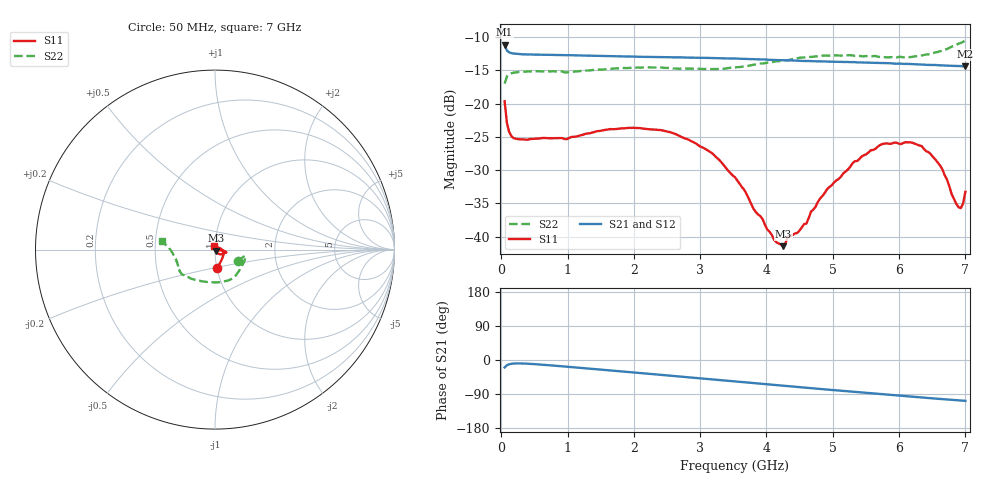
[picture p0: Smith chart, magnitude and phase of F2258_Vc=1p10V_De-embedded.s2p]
! Integrated Device Technology
! Corporate Headquarters
! 6024 Silver Creek Valley Road
! San Jose, CA 95138  USA
! Phone:  1-408-284-8200
! Toll Free:  1-800-223-1366
! Webpage:  http://www.idt.com/
! Timing and RF Division
! 515 Groton Road, Suite 102
! Westford, MA 01886-6024
! Device:  F2258
! Description: Voltage Variable RF Attenuator
! Frequency:  50.0 -  6000.00 MHz
! Package:  3x3 mm Thin QFN Plastic Package: 16 pin
! Ports:  2 RF, 2 DC
!  Pin  1  = NC
!  Pin  2  = NC
!  Pin  3  = RF2  = Port 2
!  Pin  4  = GND
!  Pin  5  = Vdd
!  Pin  6  = NC
!  Pin  7  = VCTRL
!  Pin  8  = NC
!  Pin  9  = GND
!  Pin 10  = RF1  = Port 1
!  Pin 11  = NC
!  Pin 12  = NC
!  Pin 13  = NC
!  Pin 14  = NC
!  Pin 15  = NC
!  Pin 16  = NC
! Vcntrl:  1.100 Volts
! Vdd:  +3.300 Volts
! Current:  1.162 mA
! Data:  The device was measured on a the F2258 evaluation board which has
!  individual transmission lines to the RF pins.  Data was collected
!  using a calibrated network analyzer.  The evaluation board was
!  de-embedded using a TRL calibration technique.
!  The reference plane is the edge of the package pin.
! Misc:  SN 10
!  Action Tracker AT0285
! Date Measured:  2014-12-10
! Date:  2016-01-13  MJV
! Note:
!  Integrated Device Technology supplies this data as a sample of measured
!  data at the package pin for this product.  Your particular data for this
!  product may vary.
!  Data was taken at 25 degrees C.
!  Integrated Device Technology reserves the right to change this data at anytime.
!Freq_(GHz)  S11M_(dB)  S11P_(deg)  S21M_(dB)  S21P_(deg)  S12M_(dB)  S12P_(deg)  S22M_(dB)  S22P_(deg)
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# GHz S dB R 50
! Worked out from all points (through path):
!   201 points, 50 MHz to 7 GHz, reference 50 ohm
!   highest |S21| = -11.14 dB at 50 MHz (marker M1); lowest = -14.4 dB at 7 GHz (marker M2)
!   group delay of S21, straight-line fit = 41.6 ps
!   lowest |S11| = -41.4 dB at 4.255 GHz (marker M3), VSWR 1.02, Z = 50.5 - j0.664 ohm
!   |S11| at or under -10 dB: start of sweep to end of sweep
!   |S22| runs from -17.0 to -10.5 dB; largest |S21 - S12| = 0.0014
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0.05  -19.62 -83.7  -11.14 -19.6  -11.13 -19.5  -16.98 -27.5
0.08475  -22.90 -61.4  -12.00 -13.9  -11.98 -13.9  -15.90 -15.4
0.189  -25.19 -31.2  -12.47 -9.3  -12.45 -9.3  -15.33 -11.1
1.2315  -24.67 -17.5  -12.77 -21.3  -12.75 -21.3  -15.04 -37.9
1.9265  -23.63 -14.3  -12.90 -31.8  -12.90 -31.8  -14.62 -55.5
2.37825  -23.96 -11.6  -12.98 -38.7  -12.99 -38.7  -14.55 -67.1
3.07325  -26.77 -8.1  -13.10 -49.6  -13.12 -49.6  -14.78 -89.5
3.525  -31.07 -8.1  -13.20 -56.8  -13.22 -56.7  -14.56 -107.3
4.11575  -40.48 -32.1  -13.43 -65.9  -13.38 -66.0  -13.68 -127.8
4.25475  -41.44 -50.8  -13.46 -68.0  -13.43 -68.1  -13.48 -131.1
4.32425  -40.00 -56.6  -13.48 -69.1  -13.44 -69.2  -13.47 -133.2
4.60225  -38.03 -67.0  -13.58 -73.3  -13.54 -73.3  -12.96 -139.0
4.7065  -35.92 -62.2  -13.61 -74.9  -13.55 -74.9  -12.94 -140.9
4.915  -32.85 -56.8  -13.66 -78.0  -13.61 -78.1  -12.77 -144.0
5.332  -28.65 -42.2  -13.75 -84.2  -13.74 -84.2  -12.82 -150.0
5.85325  -26.04 -26.6  -13.91 -91.7  -13.89 -91.8  -13.01 -159.8
6.20075  -25.88 -17.1  -14.05 -96.9  -14.03 -96.9  -12.96 -168.3
6.47875  -27.60 -4.0  -14.17 -100.8  -14.13 -100.8  -12.48 -175.6
6.6525  -29.86 10.0  -14.24 -103.2  -14.21 -103.2  -12.01 179.3
6.89575  -35.57 69.9  -14.34 -106.5  -14.33 -106.5  -10.97 173.4
6.96525  -35.03 98.3  -14.39 -107.4  -14.34 -107.5  -10.70 171.9
7  -33.25 110.1  -14.40 -107.8  -14.38 -107.9  -10.49 171.2
